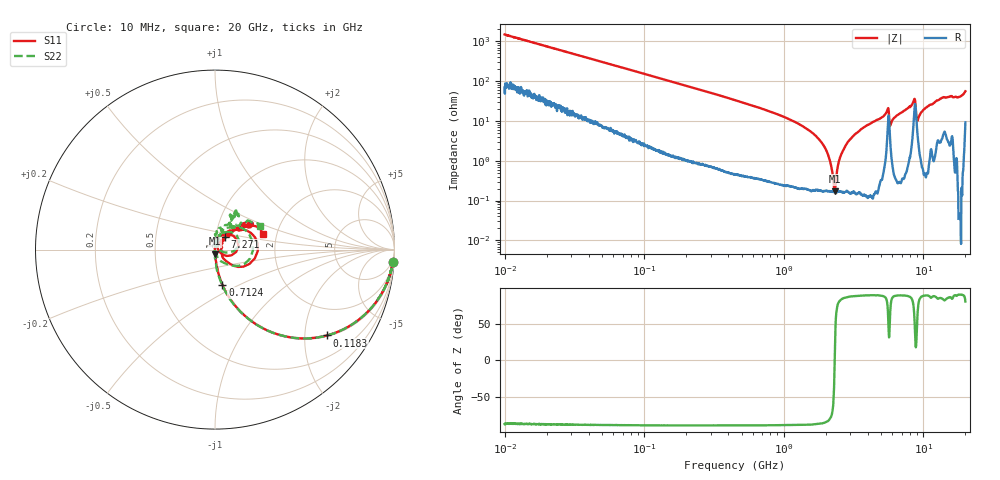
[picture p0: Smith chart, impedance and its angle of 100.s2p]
!Keysight Technologies,P5008B,MY61100088,A.16.20.02
!Date: Friday, August 30, 2024 13:27:41
!Correction: S11(C  2-Port  )
!S21(C  2-Port  )
!S12(C  2-Port  )
!S22(C  2-Port  )
!S2P File: Measurements: S11, S21, S12, S22:Log Frequency Sweep
# Hz S  MA  R 50
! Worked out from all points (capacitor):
!   1601 points, 10 MHz to 20 GHz, reference 50 ohm
!   read as one part in series: C = 10.7 pF near 10.39 MHz
!   lowest |Z| = 172 mohm at 2.314 GHz (marker M1)
!   series resonance near 2.315 GHz, so ESL is about 440 pH
!   S11 on the Smith chart (normalised r, x): 10 MHz: 2, -30; 118.3 MHz: 1.03, -2.59; 712.4 MHz: 1.00, -0.41; 7.271 GHz: 1.10, +0.16; 20 GHz: 1.68, +0.33
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1e7  0.995 -3.8  0.0668 83.5  0.06682 83.5  0.9945 -3.8
3.555162e7  0.9671 -13.2  0.2273 75.1  0.2273 75.1  0.967 -13.2
1.182591e8  0.7872 -37.4  0.6055 51.8  0.6053 51.8  0.7874 -37.4
1.263918e8  0.7674 -39.2  0.6304 50.0  0.6301 50.0  0.7676 -39.3
4.472136e8  0.3201 -70.9  0.9432 18.2  0.9428 18.2  0.3201 -71.2
7.123658e8  0.2006 -78.2  0.9767 10.8  0.9764 10.8  0.2005 -78.5
1.589917e9  0.06614 -85.4  0.9963 2.1  0.9959 2.1  0.06632 -87.4
2.313997e9  0.02344 -86.3  0.9984 -1.4  0.998 -1.4  0.02443 -87.2
2.655791e9  0.01039 -86.5  0.9987 -2.7  0.9984 -2.7  0.01187 -79.7
2.920497e9  0.001431 33.8  0.999 -3.6  0.9985 -3.6  0.002658 -8.7
3.196366e9  0.0106 90.4  0.9991 -4.5  0.9987 -4.6  0.01092 58.2
3.633803e9  0.02602 83.6  0.9989 -5.9  0.9985 -6.0  0.02446 75.8
5.467537e9  0.09796 58.2  0.973 -13.6  0.9726 -13.7  0.1005 65.9
5.652411e9  0.1189 -6.1  0.8808 -9.7  0.8806 -9.7  0.1292 7.0
6.012494e9  0.02732 53.0  0.9944 -10.7  0.9942 -10.7  0.02967 67.6
7.27077e9  0.09083 53.1  0.9955 -15.8  0.9951 -15.9  0.08681 87.9
8.626876e9  0.233 17.3  0.833 -23.2  0.8329 -23.3  0.2092 22.7
9.220141e9  0.0504 -38.9  0.9772 -14.7  0.9768 -14.9  0.02331 -71.3
9.531902e9  0.03426 2.6  0.9923 -17.1  0.9918 -17.2  0.01081 84.3
1.033363e10  0.06858 47.4  0.9977 -20.9  0.9971 -21.0  0.06544 78.1
1.27966e10  0.1871 40.9  0.9601 -27.9  0.9596 -28.0  0.1752 60.0
2e10  0.2803 18.5  0.8807 -48.2  0.8803 -48.4  0.2839 27.9
